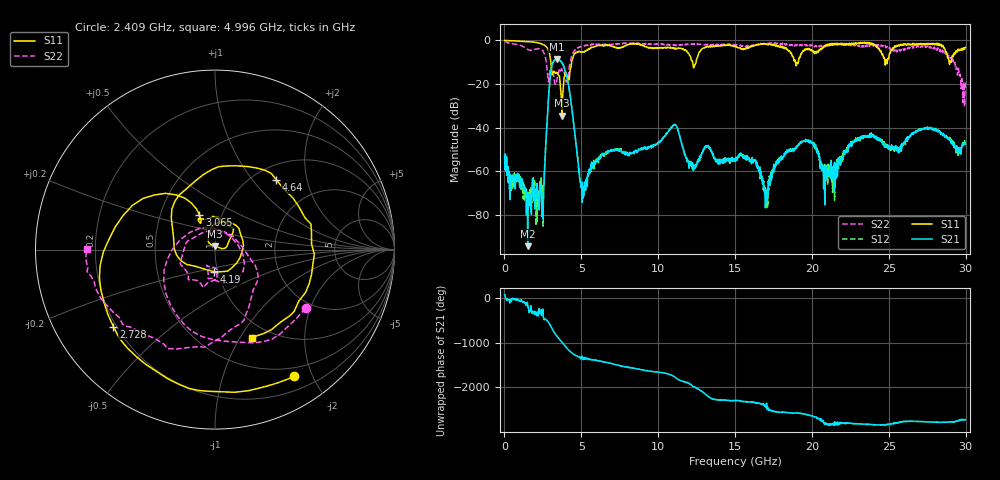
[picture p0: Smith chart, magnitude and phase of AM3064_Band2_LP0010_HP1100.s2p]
# Hz S DB R 50.0
!freq dBS11 angS11 dBS21 angS21 dBS12 angS12 dBS22 angS22
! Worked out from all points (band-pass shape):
!   1600 points, 10 MHz to 29.98 GHz, reference 50 ohm
!   highest |S21| = -8.53 dB at 3.403 GHz (marker M1); lowest = -94.4 dB at 1.51 GHz (marker M2)
!   |S21| within 3 dB of the highest: 3.09 GHz to 3.833 GHz (743.2 MHz wide, 21.5 % of centre)
!   lowest |S11| = -34.5 dB at 3.74 GHz (marker M3), VSWR 1.04, Z = 50.1 + j1.89 ohm
!   |S11| at or under -10 dB: 3.016 GHz to 4.368 GHz (1.352 GHz wide, 36.6 % of centre); 12.24 GHz to 12.46 GHz (220.4 MHz wide, 1.78 % of centre); 18.93 GHz to 19.11 GHz (181.6 MHz wide, 0.955 % of centre)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
!   |S22| runs from -30.4 to -0.2 dB; largest |S21 - S12| = 0.011
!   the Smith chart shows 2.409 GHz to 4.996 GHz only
!   S11 on the Smith chart (normalised r, x): 2.409 GHz: 0.38, -1.74; 2.728 GHz: 0.19, -0.33; 3.065 GHz: 0.78, +0.32; 4.19 GHz: 0.96, -0.24; 4.64 GHz: 1.26, +1.33; 4.996 GHz: 0.82, -1.12
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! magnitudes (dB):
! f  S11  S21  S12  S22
! 10 MHz  0.0  -53.2  -52.2  -0.2
! 1.51 GHz  -0.6  -94.4  -80.5  -4.2
! 2.409 GHz  -1.6  -68.3  -74.1  -4.4
! 2.728 GHz  -3.0  -42.3  -42.2  -10.3
! 3.065 GHz  -13.5  -12.3  -12.2  -15.3
! 3.403 GHz  -14.7  -8.5  -8.7  -18.6
! 3.74 GHz  -34.5  -10.4  -10.2  -13.5
! 4.19 GHz  -18.2  -21.4  -21.6  -13.7
! 4.64 GHz  -5.7  -46.2  -46.8  -4.5
! 4.996 GHz  -5.5  -67.1  -67.4  -3.0
! 5.015 GHz  -5.5  -66.9  -66.5  -2.8
! 10 GHz  -3.5  -47.0  -46.9  -1.8
! 11.09 GHz  -4.1  -38.6  -38.6  -2.0
! 12.21 GHz  -9.3  -56.6  -58.8  -1.9
! 15 GHz  -2.7  -54.2  -54.3  -1.9
! 17.03 GHz  -1.7  -70.9  -70.5  -1.3
! 19.99 GHz  -4.5  -46.9  -47.2  -2.1
! 20.91 GHz  -2.2  -57.3  -59.1  -2.5
! 23.21 GHz  -1.3  -44.5  -44.1  -2.2
! 25 GHz  -8.1  -49.7  -48.5  -3.0
! 28.56 GHz  -3.1  -43.0  -43.2  -4.8
! 29.98 GHz  -3.2  -47.7  -46.9  -19.1
